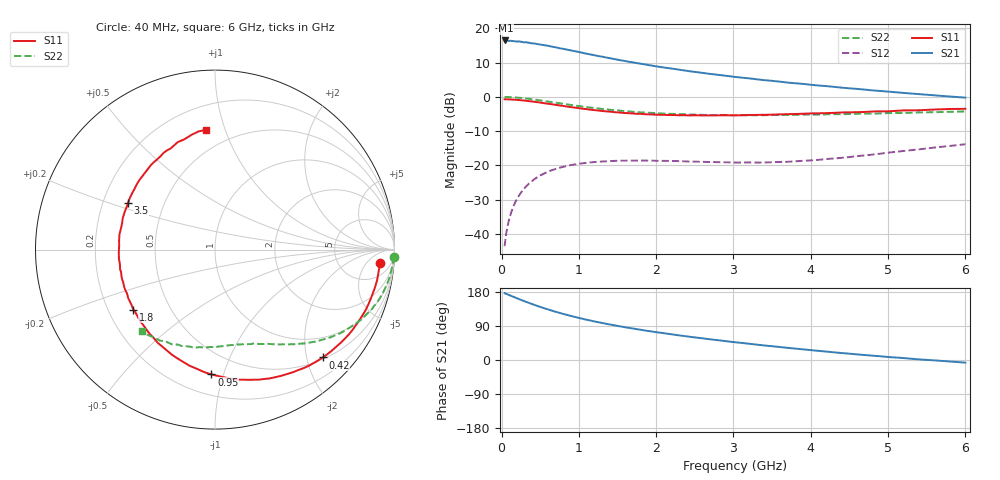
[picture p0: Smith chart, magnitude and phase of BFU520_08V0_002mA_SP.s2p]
! Filename:  P:\Prog\Test\Noise\ATS_data\Testdata_Net\03 Spar\BFU520_APG2013_37_A05_08p0V_002mA_SP_CM01_D.s2p
! Date/Time: Fri 26/Apr/2013 13:00:09
! BFU520_APG2013_37_A05_08p0V_1to20mA_SP_CM01_Bias2_R.s2p
! MDIF S-parameter v. bias file
! BFU520_APG2013_37_A05_08p0V_1to20mA_SP_CM01
! Date/time Tue Apr 23 17:06:44 2013
! VAR V_out= 8.0000
! VAR I_out= 1.9950
! VAR V_in= 0.8042
! VAR I_in= 0.0215
! Device data file deembeded for feedlines and parallel
! Original file: \03 Spar\BFU520_APG2013_37_A05_08p0V_002mA_SP_CM01_R.s2p
! Feed-files: PR047V01_250413_Feed1.s2p, PR047V01_250413_Feed2.s2p
! Parallel-file: PR047V01_250413_Par.s2p
# MHz S MA R 50
!  Freq-MHz  S11-mag  S11-arg  S21-mag  S21-arg  S12-mag  S12-arg  S22-mag  S22-arg
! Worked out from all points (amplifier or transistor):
!   98 points, 40 MHz to 6 GHz, reference 50 ohm
!   highest |S21| = 16.5 dB at 50 MHz (marker M1)
!   |S21| within 3 dB of that: start of sweep to 917.8 MHz
!   unconditionally stable (mu >= 1): 3.008 GHz to 4.924 GHz
!   at 300 MHz: K = 0.11, MSG = 21.3 dB, |S12| = -26.6 dB
!   at 1.6 GHz: K = 0.52, MSG = 14.6 dB, |S12| = -18.6 dB
!   at 6 GHz: K = 0.82, MSG = 6.8 dB, |S12| = -13.8 dB
!   S11 on the Smith chart (normalised r, x): 40 MHz: 13, -13; 420 MHz: 0.53, -2.31; 950 MHz: 0.34, -0.91; 1.8 GHz: 0.31, -0.30; 3.5 GHz: 0.31, +0.23; 6 GHz: 0.36, +0.86
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40  0.9232 -4.5  6.656 176.6  0.006585 87.1  0.9959 -2.3
50  0.9217 -5.5  6.67 175.2  0.008213 86.3  0.996 -2.8
100  0.9188 -10.9  6.553 171.4  0.01643 83.0  0.9908 -5.9
120  0.9158 -13.3  6.601 169.6  0.01964 81.8  0.9883 -7.1
180  0.9071 -19.8  6.466 164.7  0.02919 77.7  0.9799 -10.7
240  0.8947 -26.4  6.425 159.6  0.03818 73.8  0.9672 -14.1
320  0.8761 -34.8  6.266 153.3  0.04941 68.8  0.9463 -18.6
420  0.8494 -45.0  6.022 145.8  0.06202 63.1  0.9149 -23.6
550  0.8085 -57.8  5.7 136.7  0.07577 56.1  0.8709 -29.6
700  0.7645 -71.4  5.296 127.2  0.08847 49.2  0.8219 -35.6
950  0.696 -91.7  4.645 113.6  0.103 40.1  0.7461 -43.7
1050  0.6711 -98.9  4.396 108.6  0.107 37.1  0.7202 -46.6
1200  0.6404 -109.4  4.063 101.8  0.1114 33.1  0.686 -50.2
1450  0.5989 -125.0  3.583 91.8  0.1159 27.9  0.6408 -55.6
1800  0.5647 -143.6  3.05 79.8  0.1173 23.1  0.5949 -61.9
2050  0.548 -155.6  2.736 72.1  0.1161 20.8  0.5724 -66.3
2450  0.5364 -173.1  2.354 60.9  0.1133 19.3  0.5504 -72.9
3100  0.5384 163.8  1.913 45.1  0.1097 22.3  0.5391 -83.0
3500  0.5498 151.8  1.715 36.4  0.1111 26.3  0.5427 -89.4
4100  0.5755 134.6  1.464 24.1  0.1202 33.0  0.5506 -99.3
5200  0.6338 109.2  1.142 5.1  0.1619 39.2  0.5812 -118.0
6000  0.6686 94.3  0.9748 -7.0  0.2031 37.3  0.6125 -131.9
